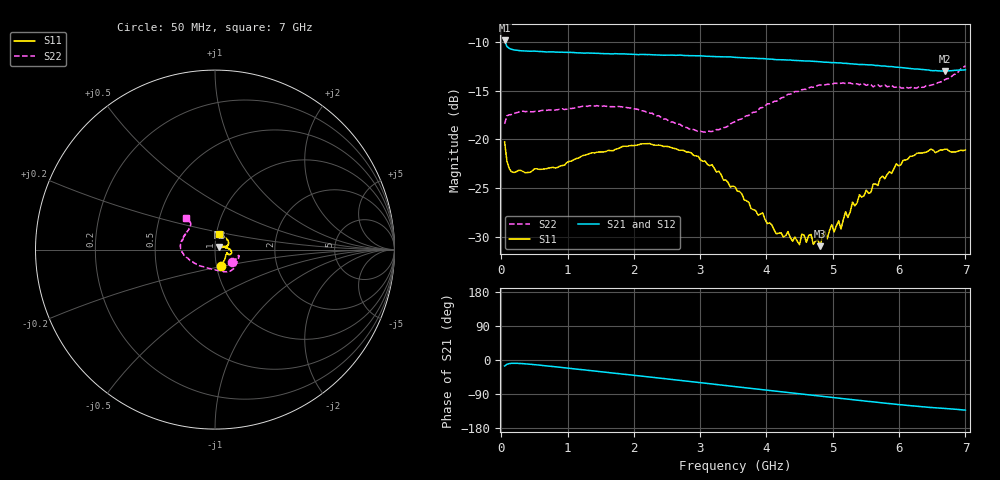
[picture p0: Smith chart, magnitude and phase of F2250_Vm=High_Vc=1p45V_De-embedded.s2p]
! Integrated Device Technology
! Corporate Headquarters
! 6024 Silver Creek Valley Road
! San Jose, CA 95138  USA
! Phone:  1-408-284-8200
! Toll Free:  1-800-223-1366
! Webpage:  http://www.idt.com/
! Timing and RF Division
! 515 Groton Road, Suite 102
! Westford, MA 01886-6024
! Device:  F2250
! Description: Voltage Variable RF Attenuator
! Frequency:  50.0 -  6000.00 MHz
! Package:  3x3 mm Thin QFN Plastic Package: 16 pin
! Ports:  2 RF, 3 DC
!  Pin  1  = GND
!  Pin  2  = NC
!  Pin  3  = RF1  = Port 1
!  Pin  4  = NC
!  Pin  5  = GND
!  Pin  6  = GND
!  Pin  7  = GND
!  Pin  8  = GND
!  Pin  9  = NC
!  Pin 10  = RF2  = Port 2
!  Pin 11  = NC
!  Pin 12  = GND
!  Pin 13  = GND
!  Pin 14  = VCNTRL
!  Pin 15  = VDD
!  Pin 16  = VMODE
! Vcntrl:  1.450 Volts
! Vmode:  +3.300 Volts
! Vdd:  +3.30  Volts
! Current:  1.329 mA
! Data:  The device was measured on a the F2250 evaluation board which has
!  individual transmission lines to the RF pins.  Data was collected
!  using a calibrated network analyzer.  The evaluation board was
!  de-embedded using a TRL calibration technique.
!  The reference plane is the edge of the package pin.
! Misc:  SN 10
!  Action Tracker AT0258
! Date Measured:  2014-11-26
! Date:  2015-10-15  MJV
! Note:
!  Integrated Device Technology supplies this data as a sample of measured
!  data at the package pin for this product.  Your particular data for this
!  product may vary.
!  Data was taken at 25 degrees C.
!  Integrated Device Technology reserves the right to change this data at anytime.
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# GHz S dB R 50
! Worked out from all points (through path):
!   201 points, 50 MHz to 7 GHz, reference 50 ohm
!   highest |S21| = -9.85 dB at 50 MHz (marker M1); lowest = -13.0 dB at 6.687 GHz (marker M2)
!   group delay of S21, straight-line fit = 52.5 ps
!   lowest |S11| = -30.9 dB at 4.811 GHz (marker M3), VSWR 1.06, Z = 52.5 + j1.52 ohm
!   |S11| at or under -10 dB: start of sweep to end of sweep
!   |S22| runs from -19.3 to -12.4 dB; largest |S21 - S12| = 0.0015
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0.05  -20.24 -70.9  -9.85 -15.9  -9.87 -15.9  -18.41 -36.3
0.08475  -22.22 -45.6  -10.47 -11.4  -10.48 -11.4  -17.57 -20.1
0.189  -23.39 -23.9  -10.81 -8.6  -10.81 -8.6  -17.34 -13.8
1.2315  -21.65 -19.3  -11.14 -25.7  -11.14 -25.7  -16.59 -41.8
2.37825  -20.57 -8.7  -11.34 -47.5  -11.35 -47.5  -17.56 -68.8
3.07325  -22.21 3.7  -11.46 -61.2  -11.46 -61.2  -19.25 -104.0
3.525  -24.86 14.1  -11.58 -70.1  -11.56 -70.2  -18.18 -132.9
4.1505  -29.69 32.5  -11.82 -82.4  -11.80 -82.5  -16.07 -161.1
4.498  -30.79 32.2  -11.92 -89.2  -11.91 -89.3  -15.06 -171.8
4.53275  -29.72 31.4  -11.94 -89.9  -11.95 -89.9  -14.90 -172.8
4.60225  -30.55 34.3  -11.96 -91.3  -11.96 -91.3  -14.87 -174.4
4.67175  -29.74 38.0  -11.97 -92.7  -11.98 -92.7  -14.63 -175.7
4.7065  -30.76 37.3  -11.99 -93.3  -11.97 -93.4  -14.64 -176.4
4.81075  -30.94 30.7  -12.04 -95.3  -12.03 -95.3  -14.41 -178.4
4.88025  -29.39 31.8  -12.08 -96.6  -12.07 -96.7  -14.40 179.5
4.915  -30.22 29.5  -12.08 -97.3  -12.09 -97.3  -14.35 178.7
5.08875  -28.34 26.0  -12.15 -100.7  -12.16 -100.7  -14.30 174.8
5.1235  -29.19 24.4  -12.15 -101.4  -12.16 -101.4  -14.24 173.8
5.29725  -26.42 18.6  -12.25 -104.6  -12.24 -104.7  -14.30 170.3
5.85325  -23.30 16.7  -12.53 -115.0  -12.49 -115.2  -14.56 155.1
6.68725  -21.01 44.8  -12.99 -127.9  -12.98 -128.0  -13.88 132.1
7  -21.08 73.8  -12.86 -132.2  -12.87 -132.4  -12.44 132.5
